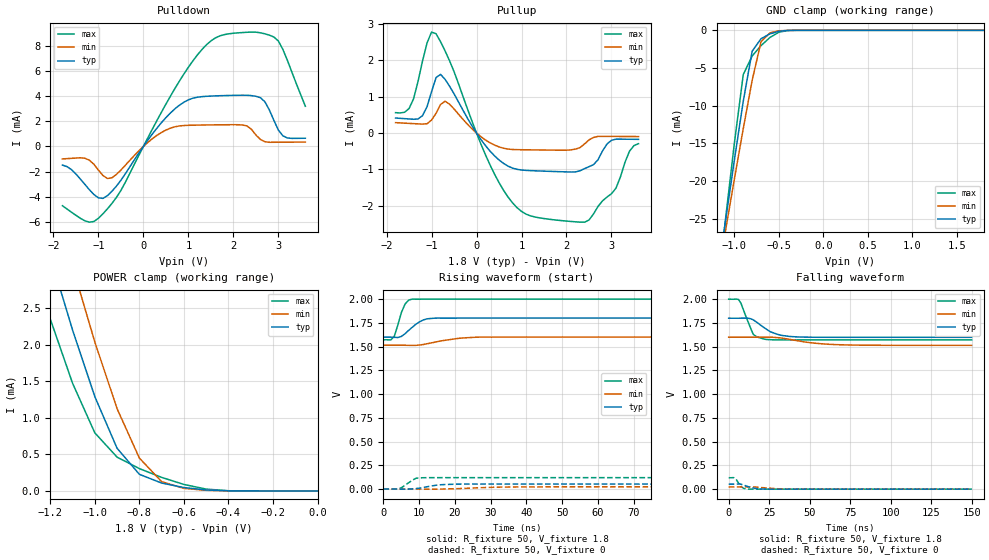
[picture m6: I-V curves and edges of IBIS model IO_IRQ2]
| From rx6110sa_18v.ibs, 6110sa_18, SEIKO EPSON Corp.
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[Model]   IO_IRQ2
Model_type 3-state
Enable Active-High
Polarity Non-Inverting
Vref=1.8
Vmeas=0.90
Rref=5000
C_comp   2.5p   2p   3p
[Temperature Range] 25   85   -40
[Voltage Range]   1.8   1.6   2.0
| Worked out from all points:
|   slope of the pulldown table from 0 to 0.27 V, typ, clamps not added: 206 ohm
|   slope of the pullup table from 0 to 0.27 V, typ, clamps not added: 599 ohm
|   GND clamp passes 1 mA (typ) near -0.68 V on its own axis
|   POWER clamp passes 1 mA (typ) near -0.96 V on its own axis
|   falling waveform, R_fixture 50, V_fixture 1.8: 20-80 % time 11.5ns typ, 21.1ns min, 5.96ns max; typ from 1.8 V to 1.6 V
|   falling waveform, R_fixture 50, V_fixture 0: 20-80 % time 6.38ns typ, NA min, 3.07ns max; typ from 0.053 V to 0 V
|   rising waveform, R_fixture 50, V_fixture 1.8: 20-80 % time 3.9ns typ, 7.86ns min, 2.21ns max; typ from 1.6 V to 1.8 V
|   rising waveform, R_fixture 50, V_fixture 0: 20-80 % time 4.97ns typ, NA min, 2.82ns max; typ from 0 V to 0.053 V
[Pullup]
-1.8V     413.3uA    286.5uA    561.7uA
-1.5V     388.1uA    266uA      674.5uA
-1.2V     479.5uA    246.2uA    1.984mA
-1V       1.135mA    356.7uA    2.776mA
-900mV    1.524mA    543.7uA    2.731mA
-700mV    1.478mA    875.9uA    2.261mA
600mV     -833.9uA   -416.9uA   -1.572mA
1V        -1.016mA   -458.5uA   -2.155mA
1.6V      -1.052mA   -467.6uA   -2.367mA
2.5V      -924.6uA   -188.6uA   -2.391mA
3V        -199.5uA   -92.46uA   -1.668mA
3.6V      -172.6uA   -96.03uA   -292uA
[Pulldown]
-1.8V     -1.483mA   -993.3uA   -4.713mA
-1.2V     -3.445mA   -1.096mA   -6.023mA
-900mV    -4.13mA    -2.311mA   -5.358mA
-700mV    -3.565mA   -2.492mA   -4.533mA
700mV     2.986mA    1.561mA    4.601mA
1.3V      3.956mA    1.701mA    7.698mA
1.7V      4.03mA     1.718mA    8.788mA
2.3V      4.068mA    1.632mA    9.073mA
2.6V      3.878mA    554.6uA    9.033mA
2.9V      2.077mA    330.7uA    8.7mA
3.1V      845.2uA    335.3uA    7.713mA
3.6V      651.4uA    347uA      3.195mA
[GND Clamp]
-1.8V     -84.94mA   -76.24mA   -100.6mA
-1.2V     -33.65mA   -33.58mA   -35.52mA
-1.1V     -25.34mA   -26.62mA   -25.12mA
-1V       -17.22mA   -19.74mA   -14.99mA
-900mV    -9.404mA   -13.04mA   -5.869mA
-800mV    -2.766mA   -6.628mA   -3.399mA
-700mV    -1.108mA   -1.501mA   -2.022mA
-600mV    -467.2uA   -331.2uA   -944.2uA
-500mV    -123.2uA   -66.32uA   -251.8uA
-400mV    -14.38uA   -8.214uA   -22.27uA
1.8V      25.75pA    24.39nA    13.19pA
[POWER Clamp]
-1.8V     9.515mA    10.63mA    8.378mA
-1.3V     4.242mA    5.194mA    3.317mA
-1.2V     3.21mA     4.128mA    2.351mA
-1.1V     2.201mA    3.07mA     1.473mA
-1V       1.29mA     2.036mA    794.1uA
-900mV    583.1uA    1.124mA    461.8uA
-800mV    227.2uA    449.5uA    305.5uA
-700mV    107.6uA    126.8uA    185uA
-600mV    46.57uA    34.75uA    88.82uA
-500mV    12.68uA    8.521uA    25.07uA
-400mV    1.719uA    1.484uA    2.421uA
0V        25.81pA    267.4pA    16.37pA
[Falling Waveform]
R_fixture=50
V_fixture=1.8
V_fixture_min=1.6
V_fixture_max=2.0
0s        1.8V       1.6V       2V
6.061ns   1.8V       1.6V       1.998V
7.576ns   1.8V       1.6V       1.958V
15.15ns   1.783V     1.6V       1.631V
18.18ns   1.747V     1.601V     1.599V
22.73ns   1.691V     1.6V       1.577V
31.82ns   1.622V     1.593V     1.572V
42.42ns   1.603V     1.563V     1.572V
71.21ns   1.599V     1.519V     1.572V
150ns     1.599V     1.514V     1.572V
[Falling Waveform]
R_fixture=50
V_fixture=0
V_fixture_min=0
V_fixture_max=0
0s        52.88mV    23.36mV    120.3mV
3.03ns    52.88mV    23.36mV    121.9mV
4.545ns   52.91mV    23.37mV    105.7mV
7.576ns   52.88mV    23.35mV    29.04mV
9.091ns   44.73mV    23.35mV    9.769mV
12.12ns   25.86mV    23.8mV     816.1uV
18.18ns   2.962mV    20.36mV    135.6uV
22.73ns   429uV      13.34mV    42.8uV
37.88ns   61.73uV    591uV      -2.632uV
150ns     -1.168uV   10.02uV    1.041uV
[Rising Waveform]
R_fixture=50
V_fixture=1.8
V_fixture_min=1.6
V_fixture_max=2.0
0s        1.599V     1.514V     1.572V
2.02ns    1.599V     1.514V     1.569V
3.03ns    1.597V     1.514V     1.606V
5.051ns   1.607V     1.514V     1.861V
6.061ns   1.635V     1.514V     1.948V
8.081ns   1.703V     1.512V     2V
11.11ns   1.779V     1.521V     2V
15.15ns   1.8V       1.552V     2V
26.26ns   1.8V       1.599V     2V
100ns     1.8V       1.6V       2V
[Rising Waveform]
R_fixture=50
V_fixture=0
V_fixture_min=0
V_fixture_max=0
0s        0V         0V         0V
4.04ns    -51.2uV    846.2nV    1.551mV
5.051ns   -603.2uV   13.47uV    13.98mV
8.081ns   1.622mV    34.63uV    92.57mV
9.091ns   4.633mV    -100.4uV   113.4mV
10.1ns    9.836mV    -324.2uV   118mV
15.15ns   42.22mV    -554.8uV   120.3mV
21.21ns   52.05mV    5.022mV    120.3mV
37.37ns   52.88mV    22.17mV    120.3mV
100ns     52.88mV    23.36mV    120.3mV
[Ramp]
R_load=50
dV/dt_r   3.173E-2/4.964E-9   1.402E-2/9.637E-9   7.219E-2/2.809E-9
dV/dt_f   1.205E-1/1.149E-8   5.110E-2/2.082E-8   2.570E-1/5.896E-9
|[End   IO_IRQ2
